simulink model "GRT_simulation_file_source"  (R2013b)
settings: Solver=FixedStepDiscrete  SolverMode=SingleTasking  StartTime=0.0  StopTime=inf  FixedStep=Param.Stepsize  RelTol=1e-3
InitFcn:
  | clear all; clc; close all;
  | Param  = Config_parameter();
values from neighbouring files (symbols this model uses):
  FFTLen = 2^(ceil(log(nFrmLen)/log(2)))    [DFT_FilterBank_Analysis_func.m]    (also in DFT_FilterBank_Synthesis_func.m; main_run3.m)
  nHopSize = size(in_frame_seg,1)    [DFT_FilterBank_Analysis_func.m]    (also in DFT_FilterBank_Synthesis_func.m = size(ref_out,1); main_run3.m = 16)
  nNumChs = size(ref_out,1)    [DFT_FilterBank_Analysis_func.m]    (also in DFT_FilterBank_Synthesis_func.m = size(in_frame,2); main_run3.m = 32; OLA_func.m = size(in_frame,2); PDbranchingsmooth_sm.m = size(x,1))
undefined symbols (not defined in the file or in its folder): a_dd, AFC_switch, BKBQ0201_16kHz, D, DownSample_factor, DownSamplingFactor, eta, example_hearing_aid, feedback_path, feedback_path_gain, Freq_shift, Fs, Ing01_ICanHear_Project, mu, prototype_win, step3_Online_simulink, VarAmpSwitch, VarAttackTime, VarCompressRatio, VarCompressTh, VarFs, VarKneeWidth, VarLimiterCompressRatio, VarLimiterTh, VarMaxSPL, VarMicNoiseCompressRatio, VarMicNoiseTh, VarRefGaindB, VarRefSPL, VarReleaseTime, VarSwitch, VarThdB, Wiener_switch
libraries: dspbuff3 x2, dspvision x2, dspadpt3 x1, dspsnks4 x1

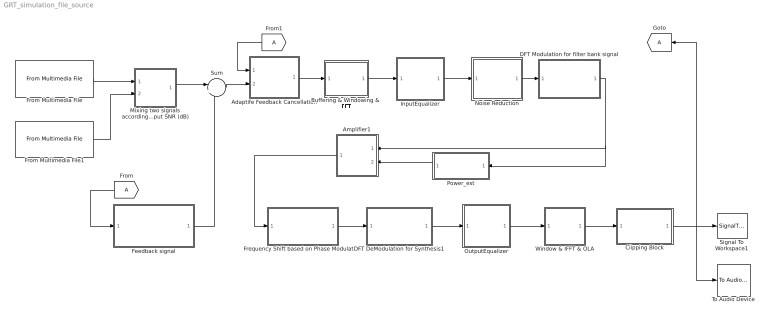
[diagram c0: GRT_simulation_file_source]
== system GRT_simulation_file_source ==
  Adaptife Feedback Cancellation : Subsystem
  Amplifier1 : Subsystem
  Buffering & Windowing &  FFT : Subsystem
  Ciipping Block : Subsystem
  DFT DeModulation for Synthesis1 : Subsystem
  DFT Modulation for filter bank signal : Subsystem
  Feedback signal : Subsystem
  Frequency Shift based on Phase Modulation : Subsystem
  From : From
  From Multimedia File : dspvision/From Multimedia File  inputFilename=D:\Ing01_ICanHear_Project\example_hearing_aid\step3_Online_simulink\BKBQ0201_16kHz.WAV  loop=on  numPlays=inf  outputStreams=Audio only  videoDataType=single  audioDataType=double  inheritSampleTime=on  userDefinedSampleTime=1/30  noAudioOutput=off  isIntensityVideo=off  fourcc=RGB  colorVideoFormat=Separate color signals  outputEOF=off  dataOrg=Column-major  audioFrameSize=Param.IO_FrameSize  computeAudioFrameSize=off  outSamplingMode=Frame based
  From Multimedia File1 : dspvision/From Multimedia File  inputFilename=D:\Ing01_ICanHear_Project\example_hearing_aid\step3_Online_simulink\speech-shaped noise_16kHz.wav  loop=on  numPlays=inf  outputStreams=Audio only  videoDataType=single  audioDataType=double  inheritSampleTime=on  userDefinedSampleTime=1/30  noAudioOutput=off  isIntensityVideo=off  fourcc=RGB  colorVideoFormat=Separate color signals  outputEOF=off  dataOrg=Column-major  audioFrameSize=Param.IO_FrameSize  computeAudioFrameSize=off  outSamplingMode=Frame based
  From1 : From
  Goto : Goto
  InputEqualizer : MATLAB Function  TreatAsAtomicUnit=on
  Mixing two signals according to an input SNR (dB) : Subsystem
  Noise Reduction : Subsystem
  OutputEqualizer : MATLAB Function  TreatAsAtomicUnit=on
  Power_est : Subsystem
  Signal To Workspace1 : SignalToWorkspace  Commented=on  VariableName=yout1
  Sum : Sum  Inputs=|++
  To Audio Device : dspsnks4/To Audio Device  deviceName=Default  inheritSampleRate=on  sampleRate=44100  deviceDatatype=Determine from input data type  autoBufferSize=on  bufferSize=4096  queueDuration=1.0  defaultOutputChannelMapping=on  outputChannelMapping=1
  Window & IFFT & OLA : Subsystem
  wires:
  Window & IFFT & OLA/1(Out1) -> Ciipping Block/1(In1)
  From Multimedia File/1 -> Mixing two signals according to an input SNR (dB)/1(In1)
  Feedback signal/1(Out1) -> Sum/2
  From/1 -> Feedback signal/1(In2)
  DFT DeModulation for Synthesis1/1(Out1) -> OutputEqualizer/1(InFreq)
  Frequency Shift based on Phase Modulation/1(Out1) -> DFT DeModulation for Synthesis1/1(In1)
  DFT Modulation for filter bank signal/1(Out1) -> Amplifier1/1(In1), Power_est/1(In1)
  Amplifier1/1(Out1) -> Frequency Shift based on Phase Modulation/1(In1)
  Noise Reduction/1(Out1) -> DFT Modulation for filter bank signal/1(In1)
  Buffering & Windowing &  FFT/1(Out1) -> InputEqualizer/1(InFreq)
  From1/1 -> Adaptife Feedback Cancellation/1(In1)
  Sum/1 -> Adaptife Feedback Cancellation/2(In2)
  Adaptife Feedback Cancellation/1(Out1) -> Buffering & Windowing &  FFT/1(In1)
  Mixing two signals according to an input SNR (dB)/1(Out1) -> Sum/1
  From Multimedia File1/1 -> Mixing two signals according to an input SNR (dB)/2(In2)
  InputEqualizer/1(OutFreqCal) -> Noise Reduction/1(In1)
  OutputEqualizer/1(OutFreqCal) -> Window & IFFT & OLA/1(In1)
  Ciipping Block/1(Out1) -> To Audio Device/1, Goto/1, Signal To Workspace1/1
  Power_est/1(Out1) -> Amplifier1/2(In2)

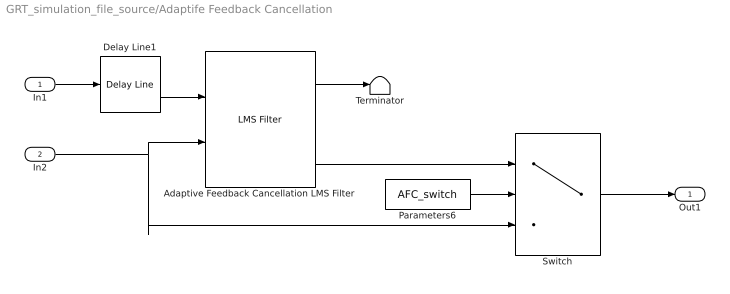
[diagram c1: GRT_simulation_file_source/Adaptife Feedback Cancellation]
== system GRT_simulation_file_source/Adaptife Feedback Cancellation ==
  In1 : Inport
  In2 : Inport  Port=2
  Adaptive Feedback Cancellation LMS Filter : dspadpt3/LMS Filter  Algo=LMS  L=128  stepflag=Dialog  mu=0.002  leakage=1.0  ic=0  Adapt=off  resetflag=None  weights=off  secondCoeffMode=User-defined  secondCoeffWordLength=2  secondCoeffFracLength=15  accum2Mode=User-defined  accum2FracLength=20  prodOutput2Mode=User-defined  prodOutput2FracLength=20  prodOutput3Mode=User-defined  prodOutput3FracLength=20  prodOutput4Mode=User-defined  prodOutput4FracLength=20  quotientMode=User-defined  quotientFracLength=20  roundingMode=Floor  overflowMode=off  addnparflag=off
  Delay Line1 : dspbuff3/Delay Line  siz=Param.IO_FrameSize  ic=0  directfeed=off  enable_output=off  hold_output=off  TreatMby1Signals=One channel
  Parameters6 : Constant  Value=AFC_switch
  Switch : Switch  Criteria=u2 > Threshold
  Terminator : Terminator
  Out1 : Outport
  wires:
  Parameters6/1 -> Switch/2
  Switch/1 -> Out1/1
  Delay Line1/1 -> Adaptive Feedback Cancellation LMS Filter/1
  Adaptive Feedback Cancellation LMS Filter/1 -> Terminator/1
  Adaptive Feedback Cancellation LMS Filter/2 -> Switch/1
  In1/1 -> Delay Line1/1
  In2/1 -> Switch/3, Adaptive Feedback Cancellation LMS Filter/2

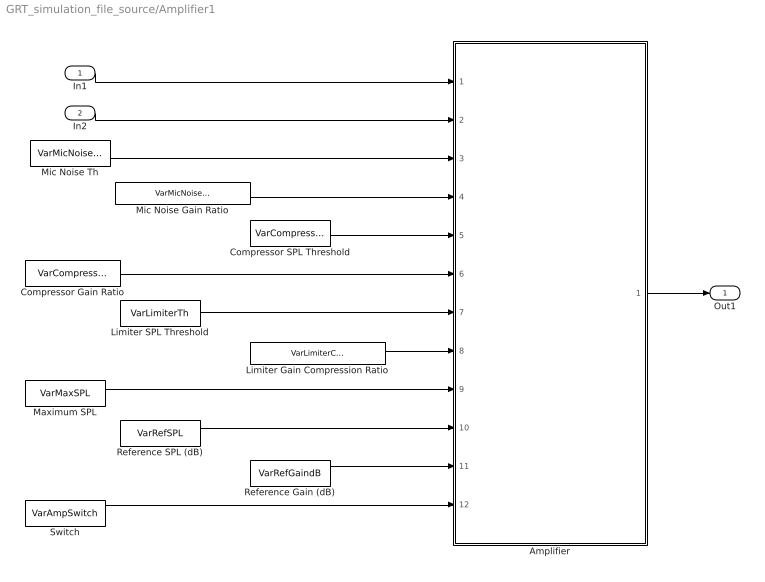
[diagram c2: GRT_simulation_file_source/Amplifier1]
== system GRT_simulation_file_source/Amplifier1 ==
  In1 : Inport
  In2 : Inport  Port=2
  Amplifier : MATLAB Function  TreatAsAtomicUnit=on
  Compressor Gain Ratio : Constant  Value=VarCompressRatio  VectorParams1D=off
  Compressor SPL Threshold : Constant  Value=VarCompressTh  VectorParams1D=off
  Limiter Gain Compression Ratio : Constant  Value=VarLimiterCompressRatio  VectorParams1D=off
  Limiter SPL Threshold : Constant  Value=VarLimiterTh  VectorParams1D=off
  Maximum SPL : Constant  Value=VarMaxSPL  VectorParams1D=off
  Mic Noise Gain Ratio : Constant  Value=VarMicNoiseCompressRatio  VectorParams1D=off
  Mic Noise Th : Constant  Value=VarMicNoiseTh  VectorParams1D=off
  Reference Gain (dB) : Constant  Value=VarRefGaindB  VectorParams1D=off
  Reference SPL (dB) : Constant  Value=VarRefSPL  VectorParams1D=off
  Switch : Constant  Value=VarAmpSwitch  VectorParams1D=off
  Out1 : Outport
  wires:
  In1/1 -> Amplifier/1(in_FBSig)
  Amplifier/1(Out_FBSig) -> Out1/1
  In2/1 -> Amplifier/2(in_EstdB)
  Compressor SPL Threshold/1 -> Amplifier/5(CT)
  Mic Noise Gain Ratio/1 -> Amplifier/4(ER)
  Mic Noise Th/1 -> Amplifier/3(ET)
  Reference Gain (dB)/1 -> Amplifier/11(G0)
  Reference SPL (dB)/1 -> Amplifier/10(L0)
  Maximum SPL/1 -> Amplifier/9(Lmax)
  Limiter Gain Compression Ratio/1 -> Amplifier/8(LR)
  Limiter SPL Threshold/1 -> Amplifier/7(LT)
  Compressor Gain Ratio/1 -> Amplifier/6(CR)
  Switch/1 -> Amplifier/12(AmpSwitch)

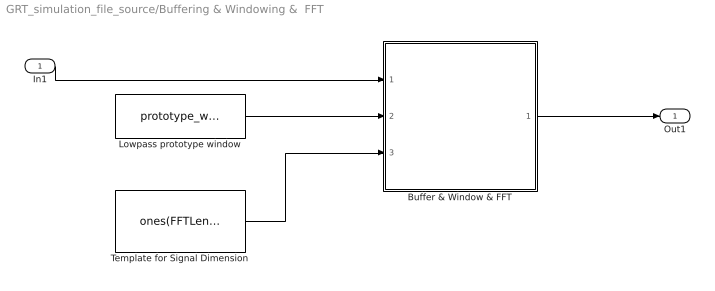
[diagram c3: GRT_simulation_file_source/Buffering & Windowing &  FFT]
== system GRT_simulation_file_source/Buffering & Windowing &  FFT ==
  In1 : Inport
  Buffer & Window & FFT : MATLAB Function  TreatAsAtomicUnit=on
  Lowpass prototype window : Constant  Value=prototype_win  VectorParams1D=off
  Template for Signal Dimension : Constant  Value=ones(FFTLen,nNumChs)  VectorParams1D=off
  Out1 : Outport
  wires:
  In1/1 -> Buffer & Window & FFT/1(in_frame_seg)
  Buffer & Window & FFT/1(FreqOut) -> Out1/1
  Template for Signal Dimension/1 -> Buffer & Window & FFT/3(ref_out)
  Lowpass prototype window/1 -> Buffer & Window & FFT/2(win)

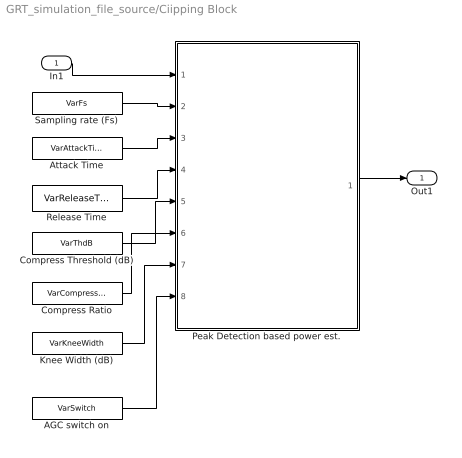
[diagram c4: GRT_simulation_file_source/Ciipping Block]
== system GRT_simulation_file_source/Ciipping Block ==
  In1 : Inport
  AGC switch on : Constant  Value=VarSwitch  VectorParams1D=off
  Attack Time : Constant  Value=VarAttackTime  VectorParams1D=off
  Compress Ratio : Constant  Value=VarCompressRatio  VectorParams1D=off
  Compress Threshold (dB) : Constant  Value=VarThdB  VectorParams1D=off
  Knee Width (dB) : Constant  Value=VarKneeWidth  VectorParams1D=off
  Peak Detection based power est. : MATLAB Function  TreatAsAtomicUnit=on
  Release Time : Constant  Value=VarReleaseTime  VectorParams1D=off
  Sampling rate (Fs) : Constant  Value=VarFs  VectorParams1D=off
  Out1 : Outport
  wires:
  In1/1 -> Peak Detection based power est./1(x)
  Peak Detection based power est./1(y) -> Out1/1
  Sampling rate (Fs)/1 -> Peak Detection based power est./2(fs)
  Attack Time/1 -> Peak Detection based power est./3(tauAttack)
  Release Time/1 -> Peak Detection based power est./4(tauRelease)
  Compress Threshold (dB)/1 -> Peak Detection based power est./5(Threshold)
  Knee Width (dB)/1 -> Peak Detection based power est./7(KneeWidth)
  Compress Ratio/1 -> Peak Detection based power est./6(ratio)
  AGC switch on/1 -> Peak Detection based power est./8(AGCSwitch)

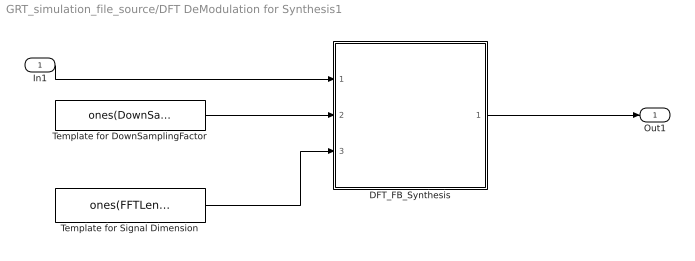
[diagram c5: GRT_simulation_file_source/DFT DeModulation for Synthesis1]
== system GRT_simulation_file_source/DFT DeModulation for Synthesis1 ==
  In1 : Inport
  DFT_FB_Synthesis : MATLAB Function  TreatAsAtomicUnit=on
  Template for DownSamplingFactor : Constant  Value=ones(DownSample_factor,1)  VectorParams1D=off
  Template for Signal Dimension : Constant  Value=ones(FFTLen,nHopSize)  VectorParams1D=off
  Out1 : Outport
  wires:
  In1/1 -> DFT_FB_Synthesis/1(FB_In)
  DFT_FB_Synthesis/1(Out_FFTSig) -> Out1/1
  Template for DownSamplingFactor/1 -> DFT_FB_Synthesis/2(ref_DownSample_factor)
  Template for Signal Dimension/1 -> DFT_FB_Synthesis/3(ref_out)

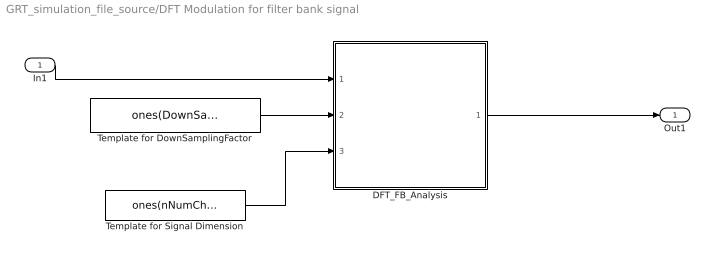
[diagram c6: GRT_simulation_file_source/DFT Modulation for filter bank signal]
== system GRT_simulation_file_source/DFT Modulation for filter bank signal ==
  In1 : Inport
  DFT_FB_Analysis : MATLAB Function  TreatAsAtomicUnit=on
  Template for DownSamplingFactor : Constant  Value=ones(DownSample_factor,1)  VectorParams1D=off
  Template for Signal Dimension : Constant  Value=ones(nNumChs,nHopSize)  VectorParams1D=off
  Out1 : Outport
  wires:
  Template for DownSamplingFactor/1 -> DFT_FB_Analysis/2(ref_DownSample_factor)
  Template for Signal Dimension/1 -> DFT_FB_Analysis/3(ref_out)
  DFT_FB_Analysis/1(FB_Out) -> Out1/1
  In1/1 -> DFT_FB_Analysis/1(in_FFTSig)

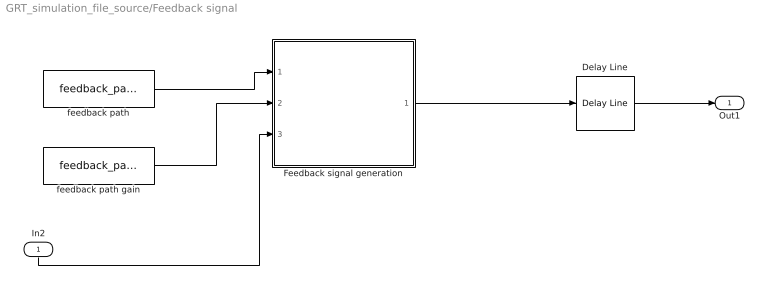
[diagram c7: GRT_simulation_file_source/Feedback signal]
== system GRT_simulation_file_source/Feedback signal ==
  In2 : Inport
  Delay Line : dspbuff3/Delay Line  siz=Param.IO_FrameSize  ic=0  directfeed=off  enable_output=off  hold_output=off  TreatMby1Signals=One channel
  Feedback signal generation : MATLAB Function  TreatAsAtomicUnit=on
  feedback path : Constant  InitFcn=|  Value=feedback_path  VectorParams1D=off
      | load('hrir_final.mat');
      | hrir=squeeze(hrir_l(13,9,:));
      | sim_ir=downsample(hrir,2);
      | feedback_path=sim_ir(10:60);
  feedback path gain : Constant  Value=feedback_path_gain  VectorParams1D=off
  Out1 : Outport
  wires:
  feedback path/1 -> Feedback signal generation/1(sim_ir)
  Feedback signal generation/1(out_sig) -> Delay Line/1
  feedback path gain/1 -> Feedback signal generation/2(feedback_path_gain)
  In2/1 -> Feedback signal generation/3(pre_receiver_output)
  Delay Line/1 -> Out1/1

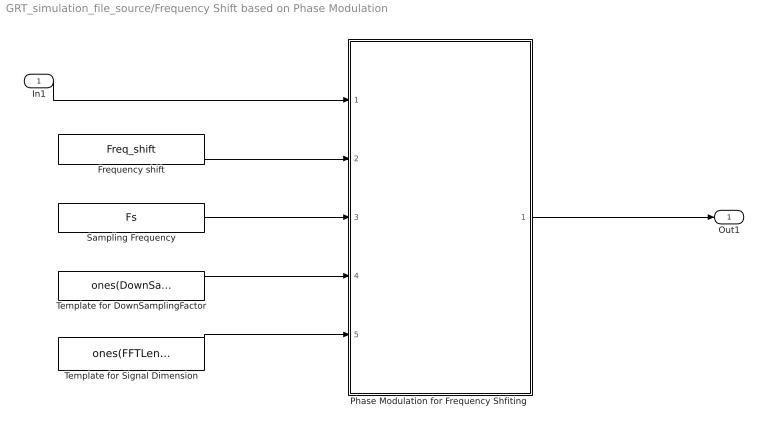
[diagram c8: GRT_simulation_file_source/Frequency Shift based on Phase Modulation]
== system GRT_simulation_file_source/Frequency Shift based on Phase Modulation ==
  In1 : Inport
  Frequency shift : Constant  Value=Freq_shift  VectorParams1D=off
  "Phase Modulation for Frequency Shfiting " : MATLAB Function  TreatAsAtomicUnit=on
  Sampling Frequency : Constant  Value=Fs  VectorParams1D=off
  Template for DownSamplingFactor : Constant  Value=ones(DownSample_factor,1)  VectorParams1D=off
  Template for Signal Dimension : Constant  Value=ones(FFTLen,nHopSize)  VectorParams1D=off
  Out1 : Outport
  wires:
  In1/1 -> "Phase Modulation for Frequency Shfiting "/1(FB_In)
  "Phase Modulation for Frequency Shfiting "/1(FreqShiftOut) -> Out1/1
  Template for DownSamplingFactor/1 -> "Phase Modulation for Frequency Shfiting "/4(ref_Downsample_factor)
  Template for Signal Dimension/1 -> "Phase Modulation for Frequency Shfiting "/5(ref_out)
  Frequency shift/1 -> "Phase Modulation for Frequency Shfiting "/2(Pm_freq)
  Sampling Frequency/1 -> "Phase Modulation for Frequency Shfiting "/3(Fs)

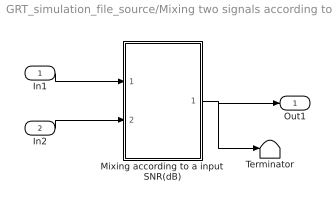
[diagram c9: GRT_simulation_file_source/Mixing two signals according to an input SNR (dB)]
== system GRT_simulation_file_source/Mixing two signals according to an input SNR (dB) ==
  In1 : Inport
  In2 : Inport  Port=2
  Mixing according to a input SNR(dB) : MATLAB Function  TreatAsAtomicUnit=on
  Terminator : Terminator
  Out1 : Outport
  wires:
  In1/1 -> Mixing according to a input SNR(dB)/1(clean_speech)
  In2/1 -> Mixing according to a input SNR(dB)/2(noise)
  Mixing according to a input SNR(dB)/1(noisy_speech) -> Out1/1, Terminator/1

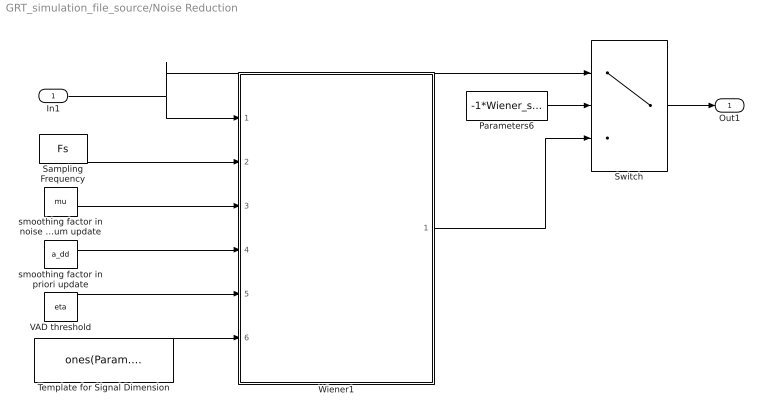
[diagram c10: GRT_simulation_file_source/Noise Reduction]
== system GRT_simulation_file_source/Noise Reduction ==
  In1 : Inport
  Parameters6 : Constant  Value=-1*Wiener_switch
  Sampling Frequency : Constant  Value=Fs  VectorParams1D=off
  Switch : Switch
  Template for Signal Dimension : Constant  Value=ones(Param.IO_FrameSize,1)  VectorParams1D=off
  VAD threshold : Constant  Value=eta  VectorParams1D=off
  Wiener1 : MATLAB Function  TreatAsAtomicUnit=on
  smoothing factor in noise spectrum update : Constant  Value=mu  VectorParams1D=off
  smoothing factor in priori update : Constant  Value=a_dd  VectorParams1D=off
  Out1 : Outport
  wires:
  In1/1 -> Switch/1, Wiener1/1(NoisyFreq)
  Sampling Frequency/1 -> Wiener1/2(Fs)
  Wiener1/1(EnhanFreq) -> Switch/3
  smoothing factor in noise spectrum update/1 -> Wiener1/3(mu)
  smoothing factor in priori update/1 -> Wiener1/4(a_dd)
  VAD threshold/1 -> Wiener1/5(eta)
  Template for Signal Dimension/1 -> Wiener1/6(ref_out)
  Switch/1 -> Out1/1
  Parameters6/1 -> Switch/2

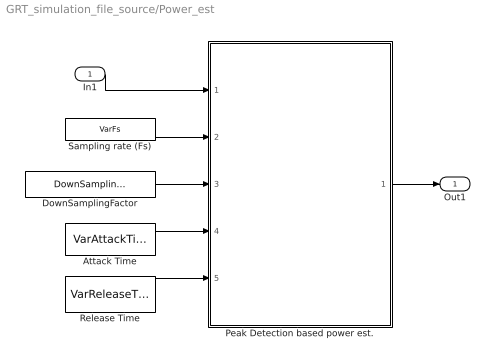
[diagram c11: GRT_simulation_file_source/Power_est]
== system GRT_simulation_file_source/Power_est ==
  In1 : Inport
  Attack Time : Constant  Value=VarAttackTime  VectorParams1D=off
  DownSamplingFactor : Constant  Value=DownSamplingFactor  VectorParams1D=off
  Peak Detection based power est. : MATLAB Function  TreatAsAtomicUnit=on
  Release Time : Constant  Value=VarReleaseTime  VectorParams1D=off
  Sampling rate (Fs) : Constant  Value=VarFs  VectorParams1D=off
  Out1 : Outport
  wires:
  In1/1 -> Peak Detection based power est./1(x)
  Peak Detection based power est./1(lg) -> Out1/1
  Sampling rate (Fs)/1 -> Peak Detection based power est./2(fs)
  Attack Time/1 -> Peak Detection based power est./4(tauAttack)
  Release Time/1 -> Peak Detection based power est./5(tauRelease)
  DownSamplingFactor/1 -> Peak Detection based power est./3(DownSamplingFactor)

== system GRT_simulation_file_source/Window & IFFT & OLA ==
  In1 : Inport
  InvFFT & Window & OLA : MATLAB Function  TreatAsAtomicUnit=on
  Template for DownSamplingFactor : Constant  Value=prototype_win  VectorParams1D=off
  Template for Signal Dimension : Constant  Value=ones(Param.IO_FrameSize,1)  VectorParams1D=off
  Out1 : Outport
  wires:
  Template for Signal Dimension/1 -> InvFFT & Window & OLA/3(ref_out)
  Template for DownSamplingFactor/1 -> InvFFT & Window & OLA/2(win)
  InvFFT & Window & OLA/1(TimeSegOut) -> Out1/1
  In1/1 -> InvFFT & Window & OLA/1(FreqIn)
